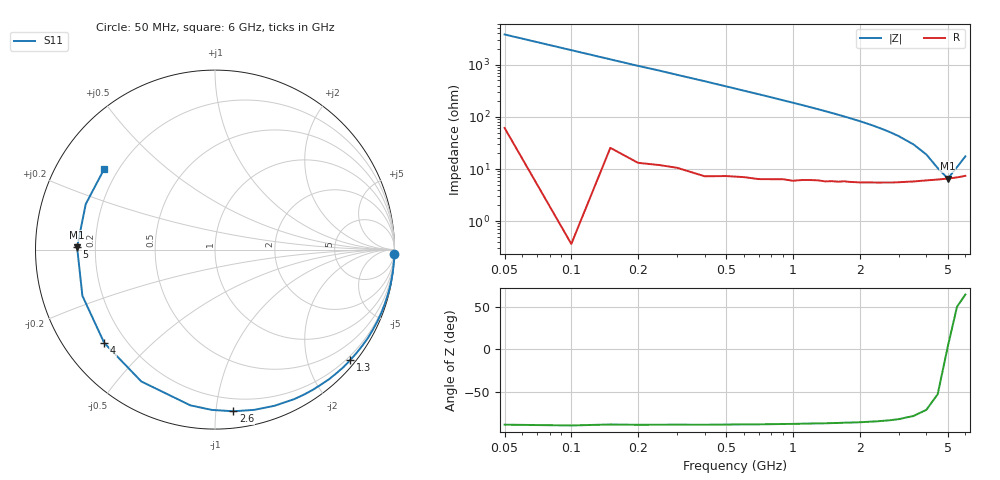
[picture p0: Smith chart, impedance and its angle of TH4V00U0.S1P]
! SIEMENS Discrete & RF Semiconductors
! BAS70
! Si Schottky Diode in SOT23
! VR = 4 V
! S-Parameters:  February  1997
# GHz  S  MA  R  50
!  f  S11
! GHz  MAG  ANG
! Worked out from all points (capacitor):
!   34 points, 50 MHz to 6 GHz, reference 50 ohm
!   read as one part to ground: C = 833 fF near 50 MHz
!   lowest |Z| = 6.56 ohm at 5 GHz (marker M1)
!   series resonance near 4.976 GHz, so ESL is about 1.2 nH
!   S11 on the Smith chart (normalised r, x): 50 MHz: 1, -76; 1.3 GHz: 0.12, -2.80; 2.6 GHz: 0.11, -1.11; 4 GHz: 0.12, -0.36; 5 GHz: 0.13, +0.01; 6 GHz: 0.15, +0.32
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0.05  0.9996 -1.5
0.1  1 -3.0
0.2  0.9986 -6.0
0.4  0.9969 -11.8
0.5  0.9951 -14.8
0.6  0.9933 -17.8
0.7  0.9917 -20.8
0.8  0.9892 -23.8
0.9  0.9863 -26.9
1  0.9842 -29.9
1.1  0.9803 -33.0
1.3  0.9731 -39.2
1.4  0.9702 -42.4
1.6  0.9617 -48.8
1.8  0.9521 -55.4
1.9  0.9475 -58.7
2  0.9427 -62.1
2.2  0.9314 -69.0
2.4  0.9194 -76.2
2.6  0.9066 -83.5
2.8  0.8933 -91.2
3  0.8785 -99.0
3.5  0.8416 -119.2
4  0.807 -139.9
4.5  0.7823 -160.8
5  0.7684 179.0
5.5  0.7635 160.6
6  0.7632 144.1
